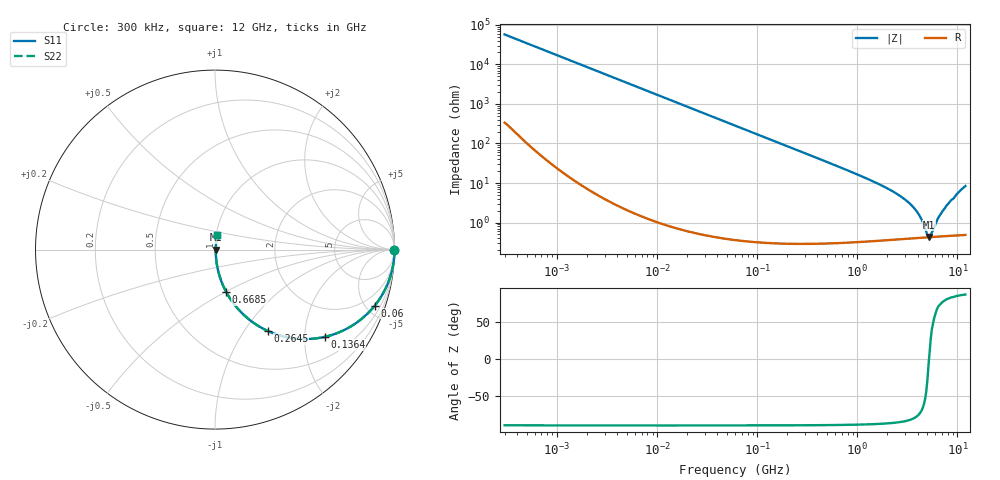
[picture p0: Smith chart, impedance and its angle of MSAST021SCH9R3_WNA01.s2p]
! MSAST021SCH9R3_WNA01  S-PARAMETER MODEL  ( General Type )
! Model Generated by TAIYO YUDEN Corporation (http://www.ty-top.com)
! Version 2.0
! TAIYO YUDEN Control No. 181101
! Copyright(c) 2015 TAIYO YUDEN CO.,LTD. All Rights Reserved.
! Product Description (link to TY-COMPAS)
! https://ds.yuden.co.jp/TYCOMPAS/or/detail?pn=MSAST021SCH9R3CWNA01&u=M
! Products Name : Multilayer Ceramic Capacitors
! Characteristics :
!  Capacitance : 9.3 pF , Rated Voltage : 25V , TCC : CH / C0H
!  Case Size : 0.25 x 0.125 / 0.0098 x 0.0049 [mm/inch] , Thickness : 0.125 / 0.0049 [mm/inch]
!  (Conditions: Temperature = 25 degC , DC Bias Current/Voltage = 0A / 0V)
! External Node Assignments :
!  1  o---| |---o  2
! GND o---------o GND
! Frequency Range : 0.3MHz  -  12000MHz  [ 401 STEP ]
# MHz S RI R 50
! Freq[MHz].  S11 Real  S11 Imag  S21 Real  S21 Imag  S12 Real  S12 Imag  S22 Real  S22 Imag
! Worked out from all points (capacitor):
!   401 points, 300 kHz to 12 GHz, reference 50 ohm
!   read as one part in series: C = 9.3 pF near 316.3 kHz
!   lowest |Z| = 430 mohm at 5.141 GHz (marker M1)
!   series resonance near 5.201 GHz, so ESL is about 100 pH
!   S11 on the Smith chart (normalised r, x): 300 kHz: open; 60 MHz: 1.01, -5.70; 136.4 MHz: 1.01, -2.51; 264.5 MHz: 1.01, -1.29; 668.5 MHz: 1.01, -0.50; 12 GHz: 1.01, +0.17
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0.3  1 -0.00175  1.34e-05 0.00175  1.34e-05 0.00175  1 -0.00175
1.769972  0.9999 -0.0103  0.000116 0.0103  0.000116 0.0103  0.9999 -0.0103
10.44266  0.9963 -0.0608  0.00375 0.0608  0.00375 0.0608  0.9963 -0.0608
26.39317  0.9767 -0.1506  0.0233 0.1506  0.0233 0.1506  0.9767 -0.1506
60  0.8902 -0.312  0.1098 0.312  0.1098 0.312  0.8902 -0.312
89.27472  0.7856 -0.4096  0.2144 0.4096  0.2144 0.4096  0.7856 -0.4096
136.3989  0.6109 -0.4863  0.3891 0.4863  0.3891 0.4863  0.6109 -0.4863
187.4445  0.4541 -0.4963  0.5459 0.4963  0.5459 0.4963  0.4541 -0.4963
264.5085  0.2948 -0.4537  0.7052 0.4537  0.7052 0.4537  0.2948 -0.4537
353.9943  0.1895 -0.3889  0.8105 0.3889  0.8105 0.3889  0.1895 -0.3889
668.5285  0.0621 -0.2354  0.9379 0.2354  0.9379 0.2354  0.0621 -0.2354
2088.533  0.00825 -0.0679  0.9918 0.0679  0.9918 0.0679  0.00825 -0.0679
2870.14  0.00551 -0.041  0.9945 0.041  0.9945 0.041  0.00551 -0.041
3642.919  0.00455 -0.0236  0.9955 0.0236  0.9955 0.0236  0.00455 -0.0236
4270.516  0.00427 -0.0128  0.9957 0.0128  0.9957 0.0128  0.00427 -0.0128
4875.354  0.00422 -0.00409  0.9958 0.00409  0.9958 0.00409  0.00422 -0.00409
5140.631  0.00424 -0.000605  0.9958 0.000605  0.9958 0.000605  0.00424 -0.000605
5420.343  0.00429 0.00228  0.9957 -0.00228  0.9957 -0.00228  0.00429 0.00228
6524.734  0.0046 0.0132  0.9954 -0.0132  0.9954 -0.0132  0.0046 0.0132
7448.838  0.00501 0.0221  0.995 -0.0221  0.995 -0.0221  0.00501 0.0221
10236.47  0.00799 0.0568  0.992 -0.0568  0.992 -0.0568  0.00799 0.0568
12000  0.0118 0.0827  0.9882 -0.0827  0.9882 -0.0827  0.0118 0.0827
